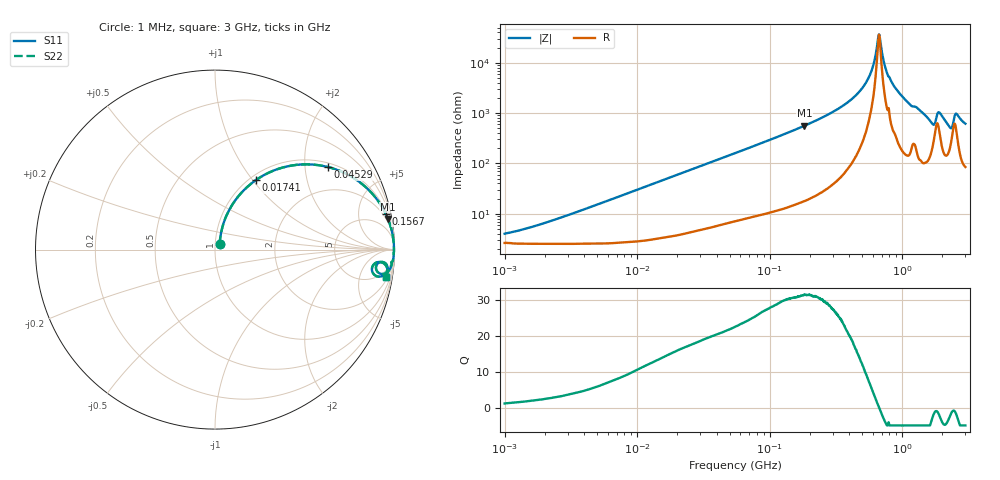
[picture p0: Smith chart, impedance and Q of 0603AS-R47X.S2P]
!s-Parameter Generated by FASTRON Sdn. Bhd.
!FASTRON P/N : 0603AS-R47X
!Keysight Technologies: E4991B_MY54100416_A.01.15
!Date created: Tue Oct 17 14:33:02 2023
!Version  : Rev01 Tue Oct 17 14:33:02 2023
!Data & Calibration Information:
!Freq	S11	S21	S12	S22
!PortZ  Port1:50+j0  Port2:50+j0
!When reading reference impedance value at option line is always used.
! Remarks : This data is being provided solely for informational purposes.
# Hz S dB R 50
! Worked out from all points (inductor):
!   1601 points, 1 MHz to 3 GHz, reference 50 ohm
!   read as one part in series: L = 478 nH near 2.524 MHz
!   highest Q = 31.5 at 182.9 MHz (marker M1), where L = 487 nH
!   self-resonance near 668.6 MHz
!   S11 on the Smith chart (normalised r, x): 1 MHz: 1.05, +0.06; 17.41 MHz: 1.07, +1.03; 45.29 MHz: 1.12, +2.64; 156.7 MHz: 1.31, +9.40; 3 GHz: 3, -12
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1000000  -28.18 47.4  -0.23 -1.7  -0.23 -1.7  -28.18 47.4
3804036  -18.91 71.1  -0.27 -6.4  -0.27 -6.4  -18.91 71.1
1.447069e7  -8.28 63.1  -0.97 -22.6  -0.97 -22.6  -8.28 63.1
1.741396e7  -6.99 59.6  -1.26 -26.5  -1.26 -26.5  -6.99 59.6
4.528757e7  -2.15 36.1  -4.59 -51.2  -4.59 -51.2  -2.15 36.1
5.477226e7  -1.61 31.3  -5.67 -56.1  -5.67 -56.1  -1.61 31.3
1.566509e8  -0.25 11.9  -13.70 -76.2  -13.70 -76.2  -0.25 11.9
1.829372e8  -0.18 10.1  -15.15 -78.1  -15.15 -78.1  -0.18 10.1
2.083556e8  -0.14 8.7  -16.43 -79.5  -16.43 -79.5  -0.14 8.7
3.523638e8  -0.05 4.2  -22.76 -83.4  -22.76 -83.4  -0.05 4.2
4.853736e8  -0.03 2.0  -29.11 -83.7  -29.11 -83.7  -0.03 2.0
5.81181e8  -0.02 0.9  -36.20 -79.5  -36.20 -79.5  -0.02 0.9
6.652545e8  -0.02 0.0  -51.06 -13.7  -51.06 -13.7  -0.02 0.0
6.855309e8  -0.02 -0.2  -48.40 44.0  -48.40 44.0  -0.02 -0.2
7.38967e8  -0.03 -0.6  -38.94 74.7  -38.94 74.7  -0.03 -0.6
7.925923e8  -0.04 -1.0  -34.58 75.5  -34.58 75.5  -0.04 -1.0
1.0437e9  -0.05 -3.0  -25.63 82.3  -25.63 82.3  -0.05 -3.0
1.67892e9  -0.50 -8.3  -16.44 64.3  -16.44 64.3  -0.50 -8.3
1.902655e9  -0.39 -4.8  -20.69 59.5  -20.69 59.5  -0.39 -4.8
2.278218e9  -0.68 -9.4  -15.18 59.9  -15.18 59.9  -0.68 -9.4
2.568929e9  -0.42 -5.1  -20.13 58.6  -20.13 58.6  -0.42 -5.1
3e9  -0.30 -8.9  -16.09 73.1  -16.09 73.1  -0.30 -8.9
